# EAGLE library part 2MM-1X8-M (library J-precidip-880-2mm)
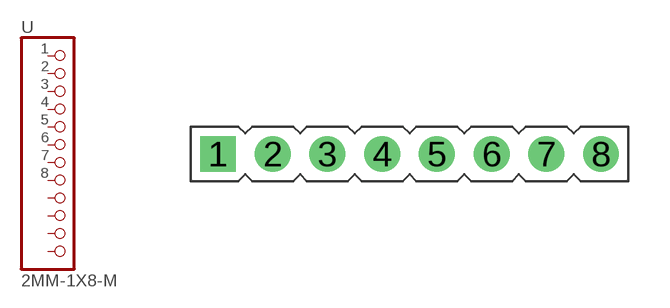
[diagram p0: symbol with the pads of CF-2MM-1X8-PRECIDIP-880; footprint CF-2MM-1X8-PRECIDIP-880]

Designator prefix -

## 2MM-1X8-M  [CF-2MM-1X8-PRECIDIP-880]
1  1  pas
2  2  pas
3  3  pas
4  4  pas
5  5  pas
6  6  pas
7  7  pas
8  8  pas

## Footprint CF-2MM-1X8-PRECIDIP-880 (pad centres in mm)
Pin Header, 1x8, 2.00mm, Through Hole Preci-Dip pn: 880-70-008-10-001101
drill 0.8 square: 1 0,0
drill 0.8: 2 2,0; 3 4,0; 4 6,0; 5 8,0; 6 10,0; 7 12,0; 8 14,0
